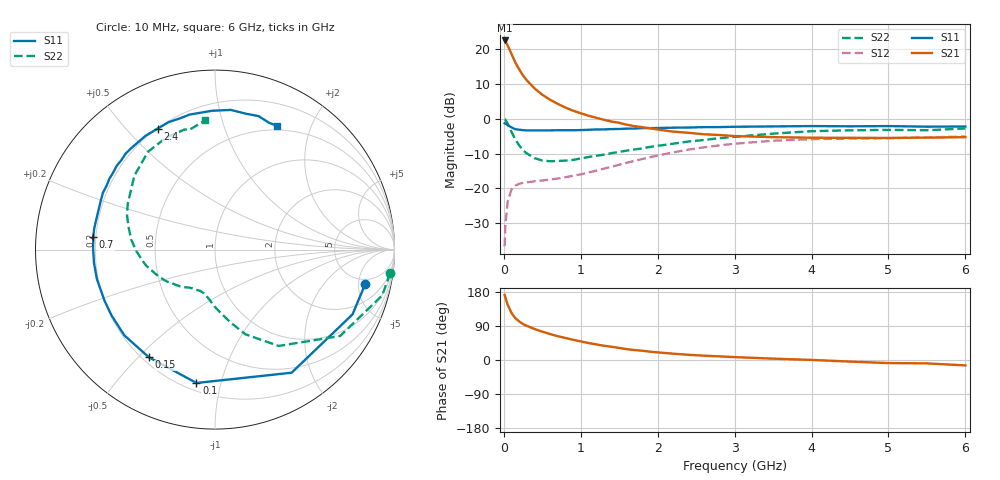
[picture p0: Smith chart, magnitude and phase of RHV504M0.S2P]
! SIEMENS Small Signal Semiconductors
! BFR106
! Si NPN RF Bipolar Junction Transistor in SOT23
! VCE = 0.5 V  IC = 4 mA
! Common Emitter S-Parameters:  August  1996
# GHz  S  MA  R  50
!  f  S11  S21  S12  S22
! GHz  MAG  ANG  MAG  ANG  MAG  ANG  MAG  ANG
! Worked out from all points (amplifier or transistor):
!   36 points, 10 MHz to 6 GHz, reference 50 ohm
!   highest |S21| = 22.4 dB at 10 MHz (marker M1)
!   |S21| within 3 dB of that: start of sweep to 82.02 MHz
!   unconditionally stable (mu >= 1): 610.8 MHz to end of sweep
!   at 250 MHz: K = 0.48, MSG = 15.4 dB, |S12| = -18.4 dB
!   at 1.4 GHz: K = 1.25, MAG = 3.4 dB, |S12| = -13.8 dB
!   at 6 GHz: K = 1.03, MAG = -1.1 dB, |S12| = -5.1 dB
!   S11 on the Smith chart (normalised r, x): 10 MHz: 4.19, -6.08; 100 MHz: 0.25, -0.84; 150 MHz: 0.23, -0.54; 700 MHz: 0.19, +0.05; 2.4 GHz: 0.20, +0.61; 6 GHz: 0.45, +1.53
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0.01  0.8589 -12.8  13.26 171.8  0.0148 84.6  0.9843 -7.7
0.02  0.847 -25.2  12.92 165.2  0.0295 76.2  0.9662 -15.3
0.05  0.8079 -58.1  11.24 145.5  0.0646 59.9  0.8475 -34.6
0.1  0.7502 -97.9  8.48 124.0  0.0964 42.7  0.6437 -56.5
0.15  0.704 -121.6  6.374 110.3  0.1096 33.4  0.5018 -70.2
0.2  0.6952 -136.7  5.084 101.7  0.1164 29.2  0.4133 -78.1
0.25  0.6834 -147.4  4.172 94.8  0.1198 26.5  0.351 -85.3
0.3  0.6782 -155.2  3.539 90.0  0.1221 25.7  0.3172 -90.4
0.4  0.6781 -166.0  2.718 81.7  0.1263 25.6  0.2715 -98.2
0.5  0.6784 -173.7  2.205 74.8  0.1296 26.9  0.2506 -104.3
0.6  0.6791 179.6  1.873 68.5  0.1337 29.1  0.2449 -109.9
0.7  0.6822 174.0  1.632 62.9  0.1383 31.5  0.2469 -115.4
0.9  0.6825 165.3  1.303 53.4  0.1514 36.3  0.2562 -124.3
1.1  0.6926 156.6  1.103 44.8  0.1686 40.6  0.2815 -133.2
1.6  0.7196 139.6  0.818 28.6  0.2333 45.6  0.3481 -154.6
2.2  0.7429 121.4  0.652 16.7  0.3284 41.4  0.4371 -178.6
2.4  0.7461 115.4  0.627 13.7  0.3595 38.5  0.4703 173.2
3.5  0.7737 91.2  0.543 3.6  0.4822 19.5  0.6099 137.4
4.5  0.7764 77.2  0.531 -4.2  0.5185 4.1  0.6808 113.4
5  0.7826 71.9  0.529 -8.1  0.5243 -1.9  0.6903 104.2
5.5  0.7679 66.9  0.534 -8.9  0.5403 -4.6  0.6823 102.1
6  0.7718 63.3  0.543 -14.3  0.5546 -11.1  0.7233 94.2
